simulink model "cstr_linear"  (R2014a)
settings: Solver=ode45  StartTime=0.0  StopTime=20  RelTol=1e-3
libraries: simulink x4

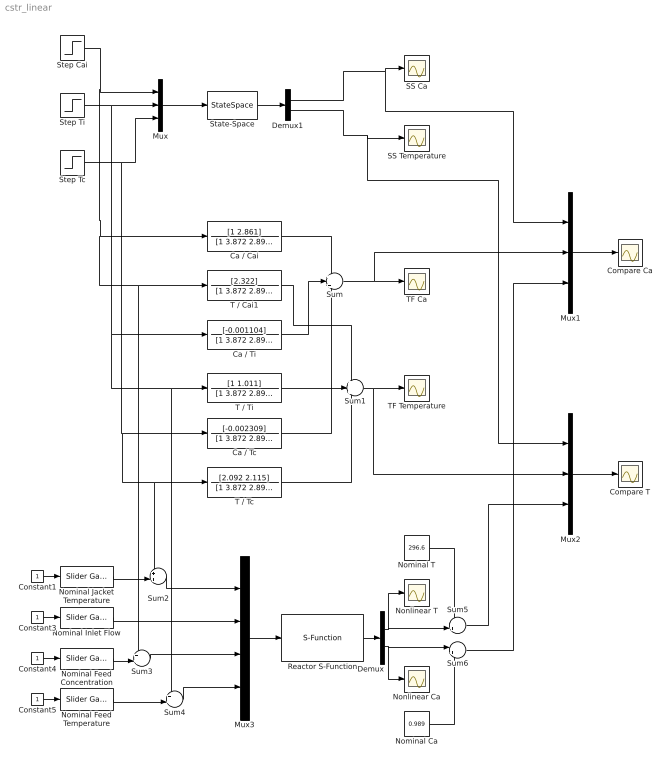
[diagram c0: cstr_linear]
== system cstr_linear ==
  Ca / Cai : TransferFcn  Numerator=[1 2.861]  Denominator=[1 3.872 2.895]
  Ca / Tc : TransferFcn  Numerator=[-0.002309]  Denominator=[1 3.872 2.895]
  Ca / Ti : TransferFcn  Numerator=[-0.001104]  Denominator=[1 3.872 2.895]
  Compare Ca : Scope
  Compare T : Scope
  Constant{1,3..5} (4 alike) : Constant
  Demux : Demux  Outputs=2
  Demux1 : Demux  Outputs=2
  Mux : Mux  Inputs=3
  Mux1 : Mux  Inputs=3
  Mux2 : Mux  Inputs=3
  Mux3 : Mux
  Nominal Ca : Constant  Value=0.989
  Nominal Feed Concentration : simulink/Math Operations/Slider Gain  low=0  gain=1  high=1
  Nominal Feed Temperature : simulink/Math Operations/Slider Gain  low=300  gain=350  high=400
  Nominal Inlet Flow : simulink/Math Operations/Slider Gain  low=0  gain=100  high=200
  Nominal Jacket Temperature : simulink/Math Operations/Slider Gain  low=250  gain=270  high=350
  Nominal T : Constant  Value=296.6
  Nonlinear Ca : Scope
  Nonlinear T : Scope
  Reactor S-Function : S-Function  FunctionName=reactor  EnableBusSupport=off
  SS Ca : Scope
  SS Temperature : Scope
  State-Space : StateSpace  A="[-1.011  -0.001104; 2.322     -2.861]"  B="[1 0 0; 0 1  2.092]"  C=[1 0; 0 1]  D=[0 0 0; 0 0 0]  X0=0
  Step Cai : Step  SampleTime=0
  Step Tc : Step  Time=10  SampleTime=0
  Step Ti : Step  Time=5  SampleTime=0
  Sum : Sum  Inputs=+++
  Sum1 : Sum  Inputs=+++
  Sum2 : Sum  Inputs=++|
  Sum3 : Sum  Inputs=++|
  Sum4 : Sum  Inputs=++|
  Sum5 : Sum  Inputs=-+|
  Sum6 : Sum  Inputs=|+-
  T / Cai1 : TransferFcn  Numerator=[2.322]  Denominator=[1 3.872 2.895]
  T / Tc : TransferFcn  Numerator=[2.092 2.115]  Denominator=[1 3.872 2.895]
  T / Ti : TransferFcn  Numerator=[1 1.011]  Denominator=[1 3.872 2.895]
  TF Ca : Scope
  TF Temperature : Scope
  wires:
  Step Cai/1 -> Mux/1, Sum3/1, T / Cai1/1, Ca / Cai/1
  Step Ti/1 -> T / Ti/1, Sum4/1, Ca / Ti/1, Mux/2
  Step Tc/1 -> Sum2/1, T / Tc/1, Ca / Tc/1, Mux/3
  Mux/1 -> State-Space/1
  Ca / Cai/1 -> Sum/1
  Ca / Ti/1 -> Sum/2
  Ca / Tc/1 -> Sum/3
  T / Cai1/1 -> Sum1/1
  T / Ti/1 -> Sum1/2
  T / Tc/1 -> Sum1/3
  Sum/1 -> Mux1/2, TF Ca/1
  Constant3/1 -> Nominal Inlet Flow/1
  Constant1/1 -> Nominal Jacket Temperature/1
  Nominal Inlet Flow/1 -> Mux3/2
  Constant4/1 -> Nominal Feed Concentration/1
  Constant5/1 -> Nominal Feed Temperature/1
  Mux3/1 -> Reactor S-Function/1
  Nominal Jacket Temperature/1 -> Sum2/2
  Sum2/1 -> Mux3/1
  Nominal Feed Concentration/1 -> Sum3/2
  Sum3/1 -> Mux3/3
  Nominal Feed Temperature/1 -> Sum4/2
  Sum4/1 -> Mux3/4
  Sum1/1 -> Mux2/2, TF Temperature/1
  Reactor S-Function/1 -> Demux/1
  State-Space/1 -> Demux1/1
  Demux1/1 -> Mux1/1, SS Ca/1
  Demux1/2 -> Mux2/1, SS Temperature/1
  Demux/1 -> Sum5/2, Nonlinear T/1
  Demux/2 -> Nonlinear Ca/1, Sum6/1
  Nominal T/1 -> Sum5/1
  Nominal Ca/1 -> Sum6/2
  Sum6/1 -> Mux1/3
  Mux1/1 -> Compare Ca/1
  Mux2/1 -> Compare T/1
  Sum5/1 -> Mux2/3
